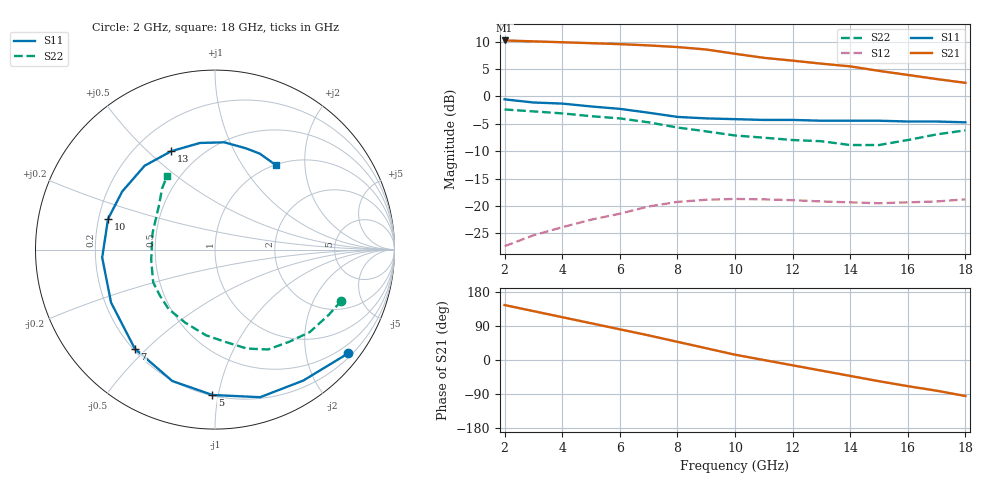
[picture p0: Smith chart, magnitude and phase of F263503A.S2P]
!ATF-26350
!S-PARAMETERS at Vds=3V  Id=10mA.  LAST UPDATED 07-22-92
# ghz s ma r 50
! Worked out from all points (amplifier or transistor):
!   17 points, 2 GHz to 18 GHz, reference 50 ohm
!   highest |S21| = 10.2 dB at 2 GHz (marker M1)
!   |S21| within 3 dB of that: start of sweep to 10.77 GHz
!   unconditionally stable (mu >= 1): 11.55 GHz to end of sweep
!   at 4 GHz: K = 0.50, MSG = 16.9 dB, |S12| = -23.9 dB
!   at 10 GHz: K = 0.88, MSG = 13.2 dB, |S12| = -18.7 dB
!   at 18 GHz: K = 1.44, MAG = 6.7 dB, |S12| = -18.8 dB
!   lowest NFmin = 1.80 dB at 6 GHz
!   S11 on the Smith chart (normalised r, x): 2 GHz: 0.29, -2.88; 5 GHz: 0.20, -0.96; 7 GHz: 0.21, -0.46; 10 GHz: 0.24, +0.13; 13 GHz: 0.35, +0.59; 18 GHz: 1.01, +1.43
2  0.94 -38.0  3.24 145.0  0.043 59.0  0.76 -22.0
3  0.88 -56.0  3.18 129.0  0.054 49.0  0.73 -30.0
4  0.86 -73.0  3.12 113.0  0.064 37.0  0.7 -41.0
5  0.81 -91.0  3.06 97.0  0.075 27.0  0.66 -51.0
6  0.77 -108.0  3 81.0  0.085 19.0  0.63 -62.0
7  0.71 -129.0  2.92 65.0  0.099 9.0  0.58 -72.0
8  0.65 -153.0  2.82 48.0  0.109 -6.0  0.52 -83.0
9  0.63 -176.0  2.68 31.0  0.114 -19.0  0.48 -96.0
10  0.62 164.0  2.45 14.0  0.116 -23.0  0.44 -112.0
11  0.61 148.0  2.25 0.0  0.115 -29.0  0.42 -128.0
12  0.61 130.0  2.12 -14.0  0.113 -36.0  0.4 -140.0
13  0.6 114.0  1.99 -28.0  0.11 -49.0  0.39 -152.0
14  0.6 98.0  1.88 -42.0  0.108 -57.0  0.36 -171.0
15  0.6 85.0  1.71 -56.0  0.106 -63.0  0.36 165.0
16  0.59 73.0  1.57 -69.0  0.108 -73.0  0.4 141.0
17  0.59 65.0  1.44 -81.0  0.11 -79.0  0.45 131.0
18  0.58 54.0  1.33 -95.0  0.115 -85.0  0.49 123.0
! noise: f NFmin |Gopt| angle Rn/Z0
6  1.8  0.49  82  0.72
8  2  0.5  118  0.52
12  2.3  0.55  -165  0.13
14  2.5  0.72  -119  0.96
